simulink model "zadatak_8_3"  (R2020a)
settings: Solver=ode23tb  StartTime=0.0  StopTime=0.06  RelTol=1e-3
undefined symbols (not defined in the file): D1, Delta
libraries: powerlib x13, sps_avr x1

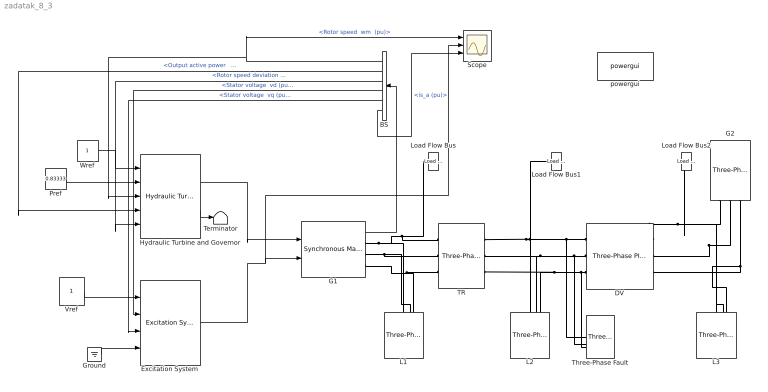
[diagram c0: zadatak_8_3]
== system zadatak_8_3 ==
  BS : BusSelector  OutputSignals="Mechanical.Rotor speed  wm  (pu),Output active power   Peo (pu),Mechanical.Rotor speed deviation  dw (pu),dq0 components.Stator voltage  vd (pu),dq0 components.Stator voltage  vq (pu),Stator current.is_a (pu)"
  DV : powerlib/Elements/Three-Phase PI Section Line  LConnTagsString=a|b|c  RConnTagsString=A|B|C  Frequency=50  Resistances=[ 0.01273 0.3864]  Inductances="[ 0.9337e-3  4.1264e-3]"  Capacitances=[12.74e-9 7.751e-9]  Length=50
  Excitation System : sps_avr/Excitation System  tr=20e-3  reg=[ 300, 0.001 ]  exc=[ 1, 0 ]  tgr=[ 0, 0 ]  damp=[ 0.001, 0.1 ]  sat=[ 0, 0 ]  lim=[ -11.5, 11.5, 0 ]  v0=[1 2.1465]
  G1 : powerlib/Machines/Synchronous Machine pu Standard  PresetModel=No  MechanicalLoad=Mechanical power Pm  ShowDetailedParameters=on  RotorType=Salient-pole  Units=per unit standard parameters  MeasurementBus=off  NominalParameters=[120e6 15.75e3 50]  Reactances1=[ 1.81, 0.3, 0.23, 1.76, 0.65, 0.25, 0.15 ]  Reactances2=[2.24 0.17 0.12 1.02 0.13 0.08]  dAxisTimeConstants=Short-circuit  qAxisTimeConstants=Short-circuit  TimeConstants1="[ 4.4849  0.0681  0.1  ]"  TimeConstants2=[ 8.0, 0.03, 1.0, 0.07 ]  TimeConstants3="[  4.49  0.0681  0.0513  ]"  TimeConstants4=[ 8.0, 0.03, 0.3371, 0.0295 ]  TimeConstants5=[ 1.01, 0.053, 0.1 ]  TimeConstants6=[ 1.3201, 0.023, 1.0, 0.07 ]  TimeConstants7=[0.012 0.003 0.003]  TimeConstants8=[ 1.3201, 0.0231, 0.3371, 0.0295 ]  StatorResistance=0.037875  Mechanical=[3 0.02056 2]  PolePairs=20  InitialConditions=[0 -77.2497 0.841643 0.841643 0.841643 -31.5874 -151.587 88.4126 2.14653]  SetSaturation=off  Saturation=[0.6404,0.7127,0.8441,0.9214,0.9956,1.082,1.19,1.316,1.457;0.7,0.7698,0.8872,0.9466,0.9969,1.046,1.1,1.151,1.201]  LoadFlowParameters=[1 0 0 0 0]  TsPowergui=0  TsBlock=-1  IterativeModel=Trapezoidal non iterative  IterativeDiscreteModel=Trapezoidal non iterative  BusType=PV  Pref=100e6  Qref=0  Qmin=-inf  Qmax=inf  PLF=0  QLF=0
  G2 : powerlib/Electrical Sources/Three-Phase Source  InternalConnection=Yg  VoltagePhases=off  Voltage=(220000)*1.5706  PhaseAngle=21.1409  Voltage_phases=[25e3 25e3 25e3]/sqrt(3)  PhaseAngles_phases=[0 -120 +120]  Frequency=50  NonIdealSource=on  SpecifyImpedance=on  Resistance=0.8929  Inductance=16.58e-3  ShortCircuitLevel=100e6  BaseVoltage=220e3  XRratio=8  BusType=swing  Pref=10e3  Qref=0  Prefabc=[10e3, 10e3, 10e3]  Qrefabc=[0, 0, 0]  Qmin=-inf  Qmax=inf
  Ground : Ground
  Hydraulic Turbine and Governor : powerlib/Machines/Hydraulic Turbine and Governor  sm="[ 10/3  0.07 ]"  gate="[  0.01  0.97518  -0.1  0.1 ]"  reg="[  0.05  1.163  0.105  0  0.01  ]"  hyd="[  0  2.67  ]"  dref=0  po=0.86016
  L1 : powerlib/Elements/Three-Phase Series RLC Load  LConnTagsString=A|B|C  Configuration=Y (grounded)  NominalVoltage=15.75e3  Vabc=[1e3 1e3 1e3]  Vabcp=[1e3 1e3 1e3]  NominalFrequency=50  UnbalancedPower=off  ActivePower=5e6  InductivePower=0  CapacitivePower=0  Pabc=[10e3 9e3 11e3]  QLabc=[100 90 110]  QCabc=[100 90 110]  Pabcp=[10e3 9e3 11e3]  QLabcp=[100 90 110]  QCabcp=[100 90 110]  Measurements=None  LoadType=constant Z
  L2 : powerlib/Elements/Three-Phase Series RLC Load  LConnTagsString=A|B|C  Configuration=Y (grounded)  NominalVoltage=220e3  Vabc=[1e3 1e3 1e3]  Vabcp=[1e3 1e3 1e3]  NominalFrequency=50  UnbalancedPower=off  ActivePower=150e6  InductivePower=50e6  CapacitivePower=0  Pabc=[10e3 9e3 11e3]  QLabc=[100 90 110]  QCabc=[100 90 110]  Pabcp=[10e3 9e3 11e3]  QLabcp=[100 90 110]  QCabcp=[100 90 110]  Measurements=None  LoadType=constant Z
  L3 : powerlib/Elements/Three-Phase Series RLC Load  LConnTagsString=A|B|C  Configuration=Y (grounded)  NominalVoltage=220e3  Vabc=[1e3 1e3 1e3]  Vabcp=[1e3 1e3 1e3]  NominalFrequency=50  UnbalancedPower=off  ActivePower=10e6  InductivePower=0  CapacitivePower=0  Pabc=[10e3 9e3 11e3]  QLabc=[100 90 110]  QCabc=[100 90 110]  Pabcp=[10e3 9e3 11e3]  QLabcp=[100 90 110]  QCabcp=[100 90 110]  Measurements=None  LoadType=constant Z
  Load Flow Bus : powerlib/Measurements/Load Flow Bus  LConnTagsString=a  Phases=single  Connectors=on one side  ID=B1  Vbase=15.75e3  Vref=1  Vangle=0  VLF=1  VLFb=1  VLFc=1  angleLF=-23.53  angleLFb=0  angleLFc=0
  Load Flow Bus1 : powerlib/Measurements/Load Flow Bus  LConnTagsString=a  Phases=single  Connectors=on one side  ID=B2  Vbase=220e3  Vref=1  Vangle=0  VLF=0.9862  VLFb=1  VLFc=1  angleLF=-0.8729  angleLFb=0  angleLFc=0
  Load Flow Bus2 : powerlib/Measurements/Load Flow Bus  LConnTagsString=a  Phases=single  Connectors=on one side  ID=B3  Vbase=220e3  Vref=1  Vangle=0  VLF=1  VLFb=1  VLFc=1  angleLF=0  angleLFb=0  angleLFc=0
  Pref : Constant  Value=0.83333
  Scope : Scope  NumInputPorts=3
  TR : powerlib/Elements/Three-Phase Transformer (Two Windings)  Winding1Connection=Delta (D1)  Winding2Connection=Yg  CoreType=Three-limb core (core-type)  SetSaturation=off  Hysteresis=off  DataFile='hysteresis'  SetInitialFlux=off  Measurements=None  UNITS=pu  NominalPower=[ 120e6 , 50 ]  Winding1=[ 15.75e3 , 0.002 , 0.08 ]  Winding2=[ 220e3 , 0.002 , 0.08 ]  Rm=500  Lm=500  L0=0.5  Saturation=[ 0,0 ; 0.0024,1.2 ; 1.0,1.52 ]  InitialFluxes=[ 0.8 , -0.8 , 0.7 ]  BreakLoop=off  DiscreteSolver=Trapezoidal iterative  DataType=off  TransfoNumber=1
  Terminator : Terminator
  Three-Phase Fault : powerlib/Elements/Three-Phase Fault  InitialStates=0  FaultA=on  FaultB=on  FaultC=on  GroundFault=off  SwitchTimes="[20e-3  70e-3]"  External=off  SwitchStatus=NaN  FaultResistance=0.001  GroundResistance=0.01  SnubberResistance=inf  SnubberCapacitance=inf  Measurements=None
  Vref : Constant
  Wref : Constant
  powergui : powerlib/powergui  Priority=1  SimulationMode=Discrete  SampleTime=1e-6  frequency=50  Iterations=100  frequencyindice=50  Pbase=100e6  ErrMax=1e-12  UnitsV=kV  UnitsW=MW  buscounter=0  FunctionMessages=off  echomessages=off  EnableUseOfTLC=off  CurrentSourceSwitches=off  DisableSnubberDevices=off  DisableRonSwitches=off  DisableVfSwitches=off  DisplayEquations=off  AutomaticDiscreteSolvers=off  SolverType=Tustin/Backward Euler (TBE)  Interpol=off  ExternalGateDelay=off  methode=off  Ts=100  x0status=blocks  SPID=on  SwTol=0  HookPort=off  NonlinearTolerance=1e-4  nMaxIteration=100  ContinueOnMaxIteration=off  RestoreLinks=warning  ResistiveCurrentMeasurement=off  Frange=[0:2:500]  Ylog=off  Xlog=on  ShowGrid=off  save=off  variable=ZData  structure=0  ZoomFFT=off  StartTime=0.0  cycles=1  DisplayStyle=1  fundamental=60  FreqAxis=off  MaxFrequency=1000  frequencyindicesteady=1  RmsSteady=1  display=off
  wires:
  G1/1 -> BS/1
  Excitation System/1 -> Scope/2, G1/2
  Hydraulic Turbine and Governor/1 -> G1/1
  Hydraulic Turbine and Governor/2 -> Terminator/1
  Wref/1 -> Hydraulic Turbine and Governor/1
  Pref/1 -> Hydraulic Turbine and Governor/2
  BS/1 -> Scope/1, Hydraulic Turbine and Governor/3  "<Rotor speed  wm  (pu)>"
  BS/2 -> Hydraulic Turbine and Governor/4  "<Output active power   Peo (pu)>"
  BS/3 -> Hydraulic Turbine and Governor/5  "<Rotor speed deviation  dw (pu)>"
  Vref/1 -> Excitation System/1
  BS/4 -> Excitation System/2  "<Stator voltage  vd (pu)>"
  BS/5 -> Excitation System/3  "<Stator voltage  vq (pu)>"
  Ground/1 -> Excitation System/4
  BS/6 -> Scope/3  "<is_a (pu)>"
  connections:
  G1/RConn1 -- L1/LConn1 -- Load Flow Bus/LConn1 -- TR/LConn1
  G1/RConn2 -- TR/LConn2 -- L1/LConn2
  G1/RConn3 -- L1/LConn3 -- TR/LConn3
  DV/LConn1 -- Three-Phase Fault/LConn1 -- Load Flow Bus1/LConn1 -- TR/RConn1 -- L2/LConn1
  DV/LConn2 -- Three-Phase Fault/LConn2 -- TR/RConn2 -- L2/LConn2
  DV/LConn3 -- Three-Phase Fault/LConn3 -- TR/RConn3 -- L2/LConn3
  G2/RConn1 -- L3/LConn1 -- Load Flow Bus2/LConn1 -- DV/RConn1
  G2/RConn2 -- DV/RConn2 -- L3/LConn2
  G2/RConn3 -- L3/LConn3 -- DV/RConn3
